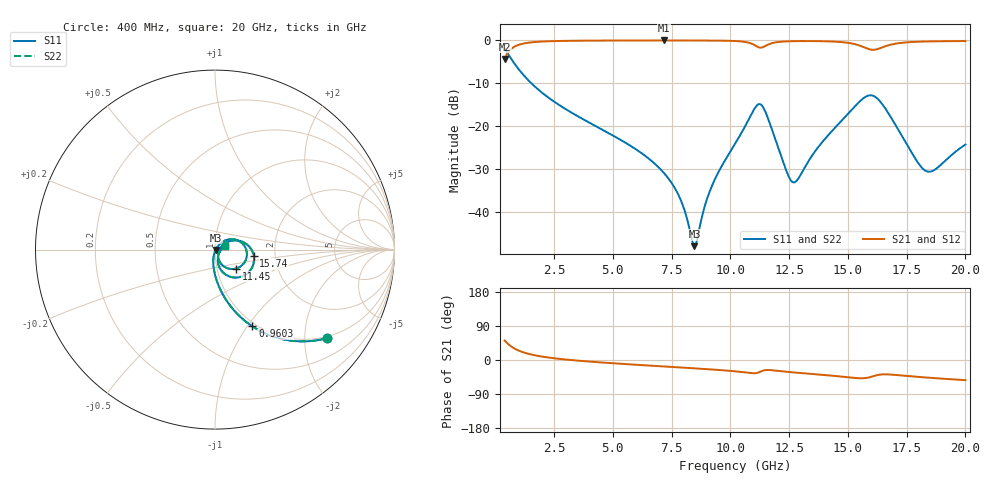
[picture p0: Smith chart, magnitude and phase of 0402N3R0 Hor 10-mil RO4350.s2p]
# GHz S MA R 50
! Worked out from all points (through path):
!   1960 points, 400 MHz to 20 GHz, reference 50 ohm
!   highest |S21| = -0.03 dB at 7.193 GHz (marker M1); lowest = -4.3 dB at 400 MHz (marker M2)
!   group delay of S21, straight-line fit = 9.85 ps
!   lowest |S11| = -47.9 dB at 8.474 GHz (marker M3), VSWR 1.01, Z = 50.4 - j0.184 ohm
!   |S11| at or under -10 dB: 1.538 GHz to end of sweep
!   |S22| runs from -47.9 to -2.0 dB; largest |S21 - S12| = 0
!   S11 on the Smith chart (normalised r, x): 400 MHz: 0.95, -2.56; 960.3 MHz: 0.96, -1.06; 11.45 GHz: 1.23, -0.27; 15.74 GHz: 1.55, -0.11; 20 GHz: 1.12, +0.05
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0.4  0.7944 -38.4  0.607 51.5  0.607 51.5  0.7944 -38.4
0.9602859  0.4758 -64.0  0.8787 25.9  0.8787 25.9  0.4758 -64.0
1.83073  0.2674 -79.0  0.9623 10.7  0.9623 10.7  0.2674 -79.0
3.671669  0.1236 -91.7  0.9904 -2.5  0.9904 -2.5  0.1236 -91.7
6.943338  0.03341 -101.5  0.9964 -16.2  0.9964 -16.2  0.03341 -101.5
7.193466  0.02825 -101.4  0.9965 -17.1  0.9965 -17.1  0.02825 -101.4
7.883818  0.01401 -96.0  0.9963 -19.7  0.9963 -19.7  0.01401 -96.0
8.474119  0.004024 -27.1  0.9956 -22.0  0.9956 -22.0  0.004024 -27.1
9.174477  0.01891 47.7  0.9938 -24.8  0.9938 -24.8  0.01891 47.7
10.205  0.06277 45.1  0.9815 -29.9  0.9815 -29.9  0.06277 45.1
11.10546  0.1715 2.1  0.8565 -34.5  0.8565 -34.5  0.1715 2.1
11.44564  0.1573 -42.2  0.8468 -27.1  0.8468 -27.1  0.1573 -42.2
12.60623  0.02291 -31.8  0.9766 -32.4  0.9766 -32.4  0.02291 -31.8
12.85636  0.02384 -0.7  0.9794 -33.7  0.9794 -33.7  0.02384 -0.7
13.46667  0.04505 29.0  0.9802 -36.8  0.9802 -36.8  0.04505 29.0
15.03747  0.1428 20.1  0.9325 -45.7  0.9325 -45.7  0.1428 20.1
15.73783  0.2189 -9.3  0.8187 -47.8  0.8187 -47.8  0.2189 -9.3
16.18806  0.2178 -41.3  0.7816 -40.9  0.7816 -40.9  0.2178 -41.3
16.73834  0.1398 -69.6  0.8775 -38.1  0.8775 -38.1  0.1398 -69.6
17.93895  0.03923 -62.5  0.9619 -44.4  0.9619 -44.4  0.03923 -62.5
18.34916  0.02994 -35.8  0.9698 -46.3  0.9698 -46.3  0.02994 -35.8
20  0.06126 20.8  0.9806 -53.2  0.9806 -53.2  0.06126 20.8
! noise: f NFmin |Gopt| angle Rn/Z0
0.4  0.001262  0.7906  3.182  0.001242
2.571  0.00506  0.6785  7.581  0.003028
4.752  0.008108  0.6392  12.93  0.00419
6.933  0.01135  0.6291  18.28  0.005601
9.104  0.01817  0.6879  23.54  0.01086
11.29  0.1243  0.936  29.08  0.4058
13.47  0.04003  0.7846  34.38  0.0349
15.64  0.1301  0.9187  39.65  0.3128
17.82  0.06754  0.8326  44.83  0.07283
20  0.04561  0.7409  49.64  0.0292
